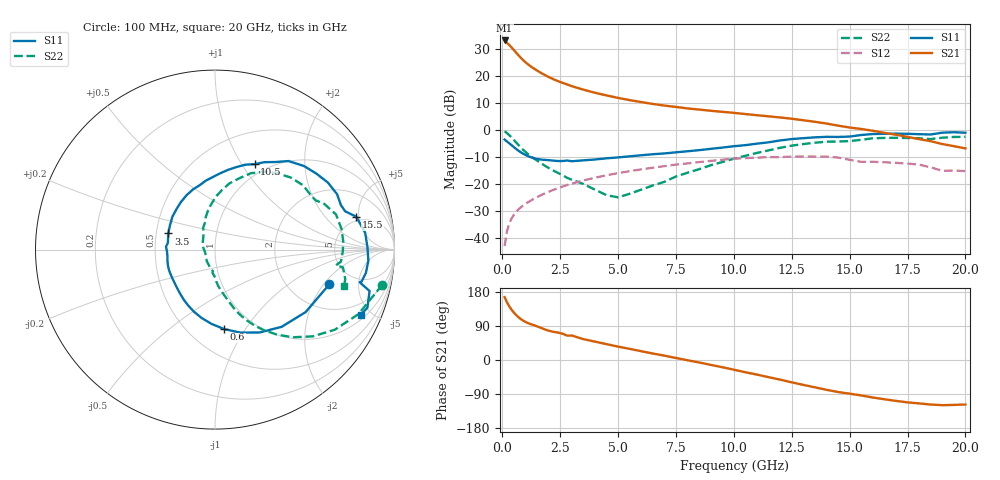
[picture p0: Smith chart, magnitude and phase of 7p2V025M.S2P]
! Infineon Technologies  Discrete & RF Semiconductors
! bfp620
! VCE =  2.0 V,  IC =  25 mA
! Common Emitter S-Parameters:  Sep 2002
# GHz  S  MA  R  50
!  f  S11  S21  S12  S22
! GHz  MAG  ANG  MAG  ANG  MAG  ANG  MAG  ANG
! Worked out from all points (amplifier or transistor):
!   59 points, 100 MHz to 20 GHz, reference 50 ohm
!   highest |S21| = 33.0 dB at 100 MHz (marker M1)
!   |S21| within 3 dB of that: start of sweep to 444.4 MHz
!   unconditionally stable (mu >= 1): 2.997 GHz to 9.911 GHz; 17.16 GHz to end of sweep
!   at 1 GHz: K = 0.74, MSG = 26.1 dB, |S12| = -27.3 dB
!   at 5.5 GHz: K = 1.04, MAG = 11.9 dB, |S12| = -15.2 dB
!   at 20 GHz: K = 1.28, MAG = 1.0 dB, |S12| = -15.2 dB
!   S11 on the Smith chart (normalised r, x): 100 MHz: 3.29, -2.29; 600 MHz: 0.73, -0.81; 3.5 GHz: 0.58, +0.11; 10.5 GHz: 0.87, +1.14; 15.5 GHz: 4.40, +4.65; 20 GHz: 1.25, -4.34
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0.1  0.6659 -16.9  44.76 165.8  0.0072 73.3  0.9522 -11.9
0.2  0.6133 -34.6  40.67 152.4  0.0135 71.1  0.8766 -24.2
0.3  0.5683 -49.2  36.92 141.6  0.0188 68.1  0.8027 -33.8
0.4  0.5245 -61.7  33.28 132.7  0.0233 65.4  0.728 -41.6
0.5  0.483 -73.1  29.8 125.2  0.0274 63.2  0.6552 -48.2
0.6  0.446 -83.4  26.63 118.6  0.031 61.5  0.5876 -53.8
0.7  0.4143 -92.7  23.84 112.8  0.0343 60.2  0.5274 -58.6
0.8  0.3878 -101.2  21.45 108.0  0.0374 59.3  0.4754 -62.6
0.9  0.3656 -108.6  19.44 103.9  0.0404 58.6  0.4312 -65.9
1.1  0.3312 -121.0  16.36 97.7  0.0461 57.8  0.3627 -70.8
1.3  0.3072 -131.1  14.16 93.1  0.0519 57.1  0.3126 -74.1
1.8  0.2818 -153.0  10.53 81.7  0.0666 55.0  0.2247 -82.3
2.2  0.2724 -166.8  8.662 74.5  0.0784 52.8  0.1788 -87.5
2.8  0.2735 176.7  6.919 64.3  0.0964 48.7  0.131 -96.2
3.5  0.2754 160.9  5.547 55.1  0.1172 43.1  0.101 -106.6
5  0.312 133.2  3.905 35.3  0.1603 29.9  0.0572 -165.1
7  0.3691 103.3  2.82 11.5  0.2154 11.3  0.1106 124.9
10.5  0.5251 65.1  1.966 -32.4  0.3027 -27.5  0.3339 83.4
13.5  0.7315 30.7  1.415 -72.1  0.3234 -63.3  0.5822 43.6
15.5  0.8082 13.1  1.043 -93.5  0.2583 -85.3  0.6591 22.8
17  0.8566 -4.1  0.817 -107.9  0.2474 -95.0  0.7158 3.9
20  0.8897 -24.1  0.458 -117.5  0.1744 -105.1  0.7472 -15.6
